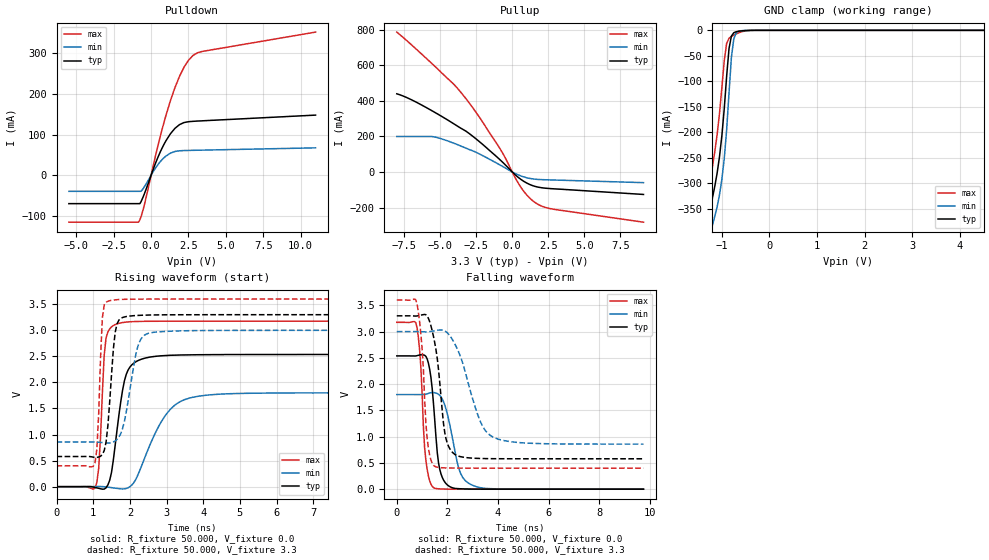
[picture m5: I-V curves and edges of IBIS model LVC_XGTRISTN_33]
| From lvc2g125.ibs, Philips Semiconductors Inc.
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|   Model LVC_XGTRISTN_33
[Model]   LVC_XGTRISTN_33
Model_type   3-state
Polarity   Non-Inverting
Enable   Active-Low
Vmeas =  1.5V
Cref  =  50.0pF
Rref  =  0.5k
Vref  =  0.0V
C_comp   3.81pF   2.87pF   5.04pF
[Model Spec]
| Note: The input and output voltage ratings may be exceeded if the input and
|   output current ratings are observed (please refer to the data sheet)
|   Subparameter   typ   min   max
| Timing Thresholds
Vmeas   1.5   1.5   1.5
|Ambient temperature:   25   85   -40
[Temperature Range]   35   95   -30
[Voltage Range]   3.3V   3.0V   3.6V
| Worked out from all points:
|   slope of the pulldown table from 0 to 0.495 V, typ, clamps not added: 10.4 ohm
|   slope of the pullup table from 0 to 0.495 V, typ, clamps not added: 14 ohm
|   GND clamp passes 1 mA (typ) near -0.58 V on its own axis
|   rising waveform, R_fixture 50.000, V_fixture 0.0: 20-80 % time 303ps typ, 754ps min, 129ps max; typ from 0 V to 2.54 V
|   rising waveform, R_fixture 50.000, V_fixture 3.3: 20-80 % time 175ps typ, 315ps min, 109ps max; typ from 0.578 V to 3.3 V
|   falling waveform, R_fixture 50.000, V_fixture 0.0: 20-80 % time 275ps typ, 486ps min, 214ps max; typ from 2.54 V to 0 V
|   falling waveform, R_fixture 50.000, V_fixture 3.3: 20-80 % time 372ps typ, 828ps min, 236ps max; typ from 3.3 V to 0.578 V
|Process Range   nominal   slow   fast
[Pulldown]
| voltage   I(typ)   I(min)   I(max)
-5.5V     -69.94mA   -39.64mA   -115.6mA
-800mV    -69.94mA   -39.64mA   -113.2mA
-700mV    -66.94mA   -39.64mA   -104.8mA
-450mV    -45.72mA   -28.25mA   -72.69mA
200mV     20.36mA    12.43mA    32.74mA
600mV     56.22mA    32.83mA    93.73mA
1.3V      102.5mA    54.49mA    184.4mA
1.9V      124.6mA    60.2mA     243.5mA
2.2V      129.7mA    60.76mA    265.9mA
2.8V      132.7mA    61.33mA    294.8mA
3.4V      133.9mA    61.77mA    304.6mA
11V       148mA      67.41mA    352.4mA
[Pullup]
| voltage   I(typ)   I(min)   I(max)
-8V       438.9mA    199.3mA    785.5mA
-7V       406mA      199.3mA    715.3mA
-5.4V     336.2mA    197mA      596.2mA
-4V       267.9mA    160mA      488.4mA
-3.4V     238.2mA    140.2mA    431.4mA
-2.4V     178.7mA    106.2mA    322.3mA
-1V       79.94mA    46.21mA    150.5mA
600mV     -41.78mA   -22.28mA   -85.9mA
1.4V      -76.37mA   -38.81mA   -160.4mA
2V        -88.29mA   -42.98mA   -190.5mA
2.8V      -94.37mA   -45.15mA   -208.6mA
9.1V      -126.4mA   -60.11mA   -282.2mA
[GND_clamp]
| voltage   I(typ)   I(min)   I(max)
-5.5V     -4.575A    -4.592A    -4.586A
-1.35V    -437.1mA   -484.4mA   -382.7mA
-1.3V     -392.9mA   -440.8mA   -337.7mA
-1.2V     -329.1mA   -382.3mA   -267.9mA
-1.05V    -247.5mA   -322.3mA   -162.7mA
-950mV    -153.2mA   -251mA     -59.23mA
-900mV    -90.01mA   -195.1mA   -25.5mA
-850mV    -35.64mA   -122.5mA   -15.63mA
-800mV    -11.36mA   -52.93mA   -12.04mA
-750mV    -4.705mA   -16.82mA   -9.379mA
-700mV    -2.761mA   -5.038mA   -7.035mA
5.5V      487.1pA    3.151nA    67.67pA
[Ramp]
| variable   typ   min   max
dV/dt_r   1.522V/302.462ps   1.080V/754.348ps   1.905V/129.033ps
dV/dt_f   1.633V/371.556ps   1.285V/827.583ps   1.920V/236.196ps
R_load = 50.000
[Rising Waveform]
R_fixture   = 50.000
V_fixture   = 0.0
V_fixture_min = 0.0
V_fixture_max = 0.0
| time   V(typ)   V(min)   V(max)
0s        22.73pV    942.1pV    4.407pV
1.05ns    -15.95mV   2.152mV    -27.29mV
1.15ns    -31.72mV   3.112mV    355mV
1.35ns    -22.24mV   -5.525mV   2.853V
1.6ns     800.4mV    -28.28mV   3.111V
1.9ns     2.153V     -35.05mV   3.158V
2.35ns    2.454V     454.6mV    3.172V
2.95ns    2.515V     1.348V     3.175V
3.6ns     2.529V     1.695V     3.175V
9.75ns    2.537V     1.801V     3.176V
[Rising Waveform]
R_fixture   = 50.000
V_fixture   = 3.3
V_fixture_min = 3.0
V_fixture_max = 3.6
| time   V(typ)   V(min)   V(max)
0s        578.4mV    857.7mV    400.2mV
1.05ns    560.9mV    857mV      459.8mV
1.15ns    568.5mV    853.1mV    1.406V
1.25ns    617.1mV    845.8mV    3.24V
1.4ns     1.167V     836.2mV    3.558V
1.6ns     2.964V     877.8mV    3.585V
1.8ns     3.246V     1.113V     3.594V
2.2ns     3.285V     2.65V      3.599V
2.5ns     3.293V     2.941V     3.6V
9.75ns    3.3V       3V         3.6V
[Falling Waveform]
R_fixture   = 50.000
V_fixture   = 0.0
V_fixture_min = 0.0
V_fixture_max = 0.0
| time   V(typ)   V(min)   V(max)
0s        2.537V     1.801V     3.176V
800ps     2.541V     1.8V       3.075V
950ps     2.558V     1.8V       2.331V
1.15ns    2.528V     1.809V     551.1mV
1.45ns    1.635V     1.839V     29.92mV
1.7ns     373.2mV    1.784V     5.076mV
2.15ns    35.04mV    1.095V     356.5uV
2.55ns    6.582mV    272.2mV    -9.159uV
3.2ns     919.3uV    39.85mV    -23.69uV
9.75ns    -2.074uV   -74.18uV   -62.35pV
[Falling Waveform]
R_fixture   = 50.000
V_fixture   = 3.3
V_fixture_min = 3.0
V_fixture_max = 3.6
| time   V(typ)   V(min)   V(max)
0s        3.3V       3V         3.6V
800ps     3.297V     3V         3.527V
1ns       3.318V     2.997V     2.681V
1.2ns     3.297V     2.996V     964.7mV
1.5ns     2.788V     3.016V     435.1mV
1.9ns     1.066V     3.012V     404.5mV
2.35ns    645.3mV    2.711V     400.7mV
3.3ns     584.2mV    1.291V     400.2mV
3.8ns     580.1mV    992.7mV    400.2mV
9.75ns    578.4mV    857.7mV    400.2mV
